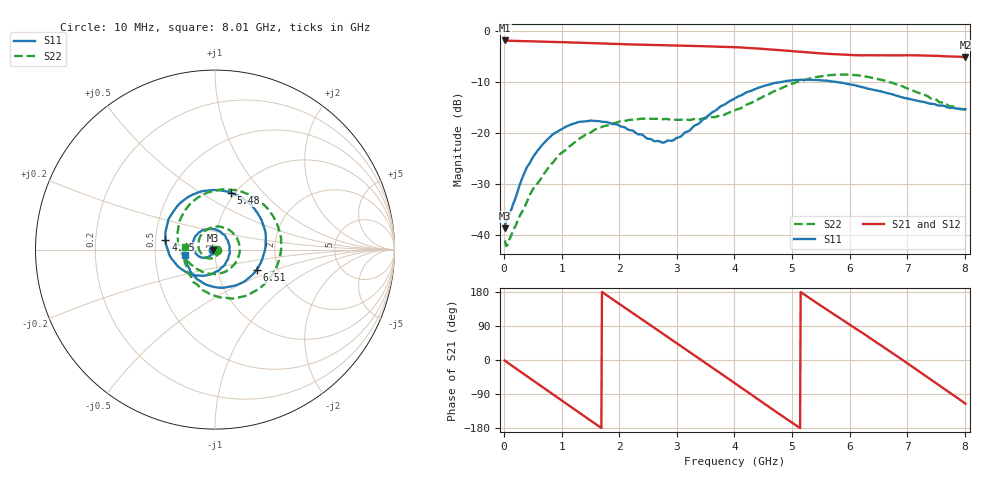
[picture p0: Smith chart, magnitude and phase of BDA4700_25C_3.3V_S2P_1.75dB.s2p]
!Agilent Technologies,E5071B,MY42404982,A.09.10
!Date: Mon Oct 20 18:03:42 2025
!Data & Calibration Information:
!Freq	S11:SOLT2(ON)	S21:SOLT2(ON)	S12:SOLT2(ON)	S22:SOLT2(ON)
# Hz S RI R 50
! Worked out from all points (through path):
!   801 points, 10 MHz to 8.01 GHz, reference 50 ohm
!   highest |S21| = -1.87 dB at 10 MHz (marker M1); lowest = -5.1 dB at 8.01 GHz (marker M2)
!   group delay of S21, straight-line fit = 288 ps
!   lowest |S11| = -38.6 dB at 10 MHz (marker M3), VSWR 1.02, Z = 48.9 - j0.196 ohm
!   |S11| at or under -10 dB: start of sweep to 4.814 GHz; 5.779 GHz to end of sweep
!   |S22| runs from -42.1 to -8.5 dB; largest |S21 - S12| = 0.0086
!   S11 on the Smith chart (normalised r, x): 10 MHz: 0.98, -0.00; 4.45 GHz: 0.56, +0.07; 5.48 GHz: 0.96, +0.68; 6.51 GHz: 1.55, -0.38; 8.01 GHz: 0.71, -0.05
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1e7  -0.0115 -0.00201  0.8058 -0.0173  0.8055 -0.0179  0.00879 -0.00106
3.3e8  -0.0227 -0.0304  0.6455 -0.4626  0.645 -0.4626  0.0159 -0.00751
7.2e8  -0.0695 -0.0453  0.175 -0.7638  0.1752 -0.7637  0.000625 -0.042
1.02e9  -0.1097 -0.0184  -0.2498 -0.7335  -0.25 -0.7336  -0.0462 -0.0461
1.35e9  -0.1227 0.0406  -0.616 -0.453  -0.6163 -0.4535  -0.0906 0.00705
1.92e9  -0.0395 0.1161  -0.6843 0.2977  -0.6845 0.2976  -0.0113 0.1249
2.32e9  0.0413 0.0884  -0.3092 0.6656  -0.3092 0.6655  0.1029 0.0901
2.68e9  0.0806 0.0218  0.1565 0.7088  0.1558 0.7082  0.1365 -0.019
3.06e9  0.0642 -0.0661  0.5667 0.4397  0.5617 0.4441  0.0729 -0.1134
3.36e9  0.00976 -0.1213  0.7053 0.084  0.7061 0.0837  -0.00739 -0.1353
3.67e9  -0.0808 -0.1449  0.633 -0.304  0.6327 -0.3059  -0.086 -0.1151
4.01e9  -0.1929 -0.1048  0.3299 -0.6086  0.3307 -0.6075  -0.1553 -0.0618
4.45e9  -0.2759 0.0556  -0.2068 -0.6368  -0.2066 -0.6386  -0.2074 0.0708
4.9e9  -0.1977 0.2559  -0.5821 -0.2698  -0.5809 -0.2731  -0.1395 0.2531
5.35e9  0.0207 0.3308  -0.57 0.2227  -0.5713 0.2197  0.0895 0.3328
5.48e9  0.0898 0.3165  -0.4978 0.3424  -0.4992 0.3406  0.1649 0.3166
6e9  0.2734 0.1235  -0.0314 0.5801  -0.0359 0.5817  0.3647 0.0814
6.51e9  0.232 -0.1132  0.4277 0.387  0.4297 0.3861  0.2761 -0.1909
6.68e9  0.1769 -0.1681  0.5232 0.2409  0.5246 0.2399  0.2012 -0.2429
7.06e9  0.0311 -0.2124  0.5579 -0.1457  0.5575 -0.1465  0.0247 -0.2655
7.46e9  -0.0983 -0.1654  0.3124 -0.4777  0.312 -0.4784  -0.1174 -0.1828
8.01e9  -0.1689 -0.0311  -0.236 -0.5019  -0.2345 -0.503  -0.1681 0.0132
